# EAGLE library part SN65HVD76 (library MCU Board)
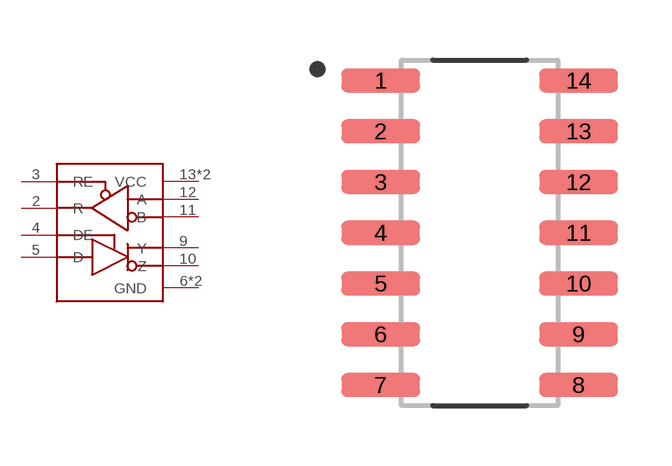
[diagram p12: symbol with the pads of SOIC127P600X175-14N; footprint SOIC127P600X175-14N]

Designator prefix U

## SN65HVD76  [SOIC127P600X175-14N]
2  R
3  RE
4  DE
5  D
6  GND
7  GND
9  Y
10  Z
11  B
12  A
13  VCC
14  VCC

## Footprint SOIC127P600X175-14N (pad centres in mm)
smd 1.97 x 0.6: 1 -2.475,3.81; 2 -2.475,2.54; 3 -2.475,1.27; 4 -2.475,0; 5 -2.475,-1.27; 6 -2.475,-2.54; 7 -2.475,-3.81; 8 2.475,-3.81; 9 2.475,-2.54; 10 2.475,-1.27; 11 2.475,0; 12 2.475,1.27; 13 2.475,2.54; 14 2.475,3.81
